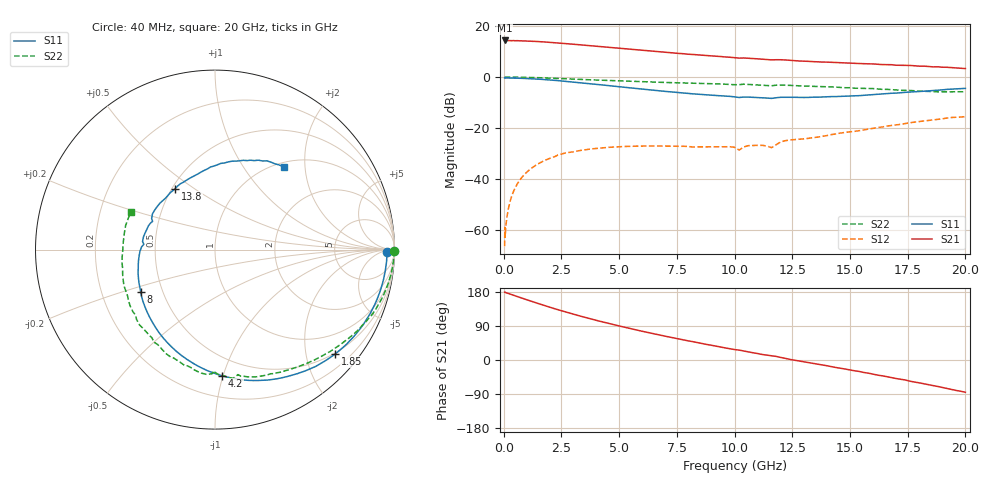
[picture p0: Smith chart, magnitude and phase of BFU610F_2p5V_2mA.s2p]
! Filename:  P:\Prog\Test\Noise\ATS_data\Testdata_Net\SplitFiles\BFU610_2W_A5_HighFreq_2.5V_2mA_D.s2p
! Date/Time: Wed 10/Aug/2011 16:55:14
! BFU610_2W_A5_HighFreq_Bias2_2.5V_1mA_10mA_R.s2p
! MDIF S-parameter v. bias file
! BFU610_2W_A5_HighFreq_2.5V_1mA_10mA
! Date/time Mon Aug 08 14:04:20 2011
! VAR V_out= 2.5010
! VAR I_out= 2.0000
! VAR V_in= 0.8679
! VAR I_in= 0.0150
! Device data file deembeded for feedlines and parallel
! Original file: \SplitFiles\BFU610_2W_A5_HighFreq_2.5V_2mA_R.s2p
! Feed-files: PR003V01_101208_Feed1.s2p, PR003V01_101208_Feed2.s2p
! Parallel-file: PR003V01_101208_Par.s2p
# MHz S MA R 50
!  Freq-MHz  S11-mag  S11-arg  S21-mag  S21-arg  S12-mag  S12-arg  S22-mag  S22-arg
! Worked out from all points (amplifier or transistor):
!   167 points, 40 MHz to 20 GHz, reference 50 ohm
!   highest |S21| = 14.3 dB at 40 MHz (marker M1)
!   |S21| within 3 dB of that: start of sweep to 4.936 GHz
!   unconditionally stable (mu >= 1): 6.71 GHz to 18.86 GHz
!   at 550 MHz: K = 0.01, MSG = 28.4 dB, |S12| = -42.5 dB
!   at 4.2 GHz: K = 0.54, MSG = 19.8 dB, |S12| = -27.8 dB
!   at 20 GHz: K = 0.91, MSG = 9.4 dB, |S12| = -15.5 dB
!   S11 on the Smith chart (normalised r, x): 40 MHz: 42, -15; 1.85 GHz: 0.48, -2.60; 4.2 GHz: 0.36, -1.00; 8 GHz: 0.38, -0.23; 13.8 GHz: 0.52, +0.42; 20 GHz: 1.08, +1.55
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40  0.9583 -0.9  5.192 178.9  0.0004908 90.4  0.9963 -0.4
50  0.9499 -1.2  5.171 179.0  0.00115 76.2  0.9968 -0.5
60  0.9594 -1.0  5.183 178.1  0.0007339 74.3  0.9971 -0.6
100  0.9593 -2.2  5.155 177.6  0.001273 89.5  0.9969 -1.0
200  0.9577 -4.5  5.147 175.6  0.002613 90.2  0.9966 -2.1
480  0.9526 -10.9  5.133 169.8  0.006556 86.2  0.9942 -5.2
1150  0.9274 -25.8  5.036 155.9  0.01572 74.6  0.9801 -12.3
1850  0.8873 -40.9  4.822 142.1  0.02412 63.9  0.9583 -19.3
2700  0.8212 -58.4  4.518 126.4  0.03281 51.8  0.9227 -27.2
3400  0.7674 -71.9  4.236 114.5  0.03705 44.2  0.8958 -33.2
4200  0.7045 -86.6  3.943 101.8  0.04096 36.3  0.8657 -39.3
5400  0.6187 -107.6  3.522 84.1  0.04398 27.2  0.8271 -48.2
6800  0.534 -130.9  3.097 65.4  0.04461 19.9  0.7881 -57.8
8000  0.4769 -150.3  2.792 50.5  0.04376 16.4  0.7576 -66.0
9400  0.4296 -172.4  2.517 34.1  0.04321 18.1  0.731 -75.8
10200  0.3973 175.7  2.344 26.1  0.03718 19.9  0.7084 -79.6
12000  0.4014 150.2  2.178 6.7  0.0538 36.8  0.6973 -93.7
13400  0.4032 128.4  2 -8.9  0.06523 30.4  0.6568 -107.2
13800  0.406 123.1  1.961 -13.0  0.06896 30.7  0.6466 -110.8
16800  0.4815 86.1  1.742 -46.5  0.1129 17.8  0.5675 -146.4
18400  0.5356 68.4  1.61 -65.5  0.1416 4.8  0.5233 -172.0
20000  0.5997 50.3  1.463 -85.2  0.1678 -12.0  0.5139 156.1
